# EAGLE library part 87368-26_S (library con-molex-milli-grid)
RECEPTACAL
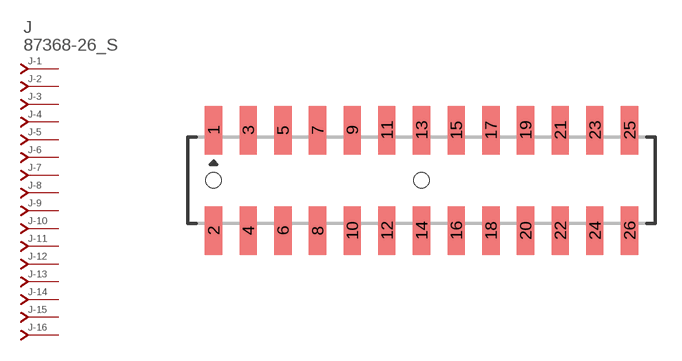
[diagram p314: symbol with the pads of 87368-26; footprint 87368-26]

Designator prefix J; gates -1=J-NV -2=J-N -3=J-N -4=J-N -5=J-N -6=J-N -7=J-N -8=J-N -9=J-N -10=J-N -11=J-N -12=J-N -13=J-N -14=J-N -15=J-N -16=J-N -17=J-N -18=J-N -19=J-N -20=J-N -21=J-N -22=J-N -23=J-N -24=J-N -25=J-N -26=J-N

## 87368-26_S  [87368-26]
1  -1:J  pas
2  -2:J  pas
3  -3:J  pas
4  -4:J  pas
5  -5:J  pas
6  -6:J  pas
7  -7:J  pas
8  -8:J  pas
9  -9:J  pas
10  -10:J  pas
11  -11:J  pas
12  -12:J  pas
13  -13:J  pas
14  -14:J  pas
15  -15:J  pas
16  -16:J  pas
17  -17:J  pas
18  -18:J  pas
19  -19:J  pas
20  -20:J  pas
21  -21:J  pas
22  -22:J  pas
23  -23:J  pas
24  -24:J  pas
25  -25:J  pas
26  -26:J  pas

## Footprint 87368-26 (pad centres in mm)
RECEPTACAL SMD Dual Row, Side Entry
smd 1 x 2.8: 1 -12,2.9; 2 -12,-2.9; 3 -10,2.9; 4 -10,-2.9; 5 -8,2.9; 6 -8,-2.9; 7 -6,2.9; 8 -6,-2.9; 9 -4,2.9; 10 -4,-2.9; 11 -2,2.9; 12 -2,-2.9; 13 0,2.9; 14 0,-2.9; 15 2,2.9; 16 2,-2.9; 17 4,2.9; 18 4,-2.9; 19 6,2.9; 20 6,-2.9; 21 8,2.9; 22 8,-2.9; 23 10,2.9; 24 10,-2.9; 25 12,2.9; 26 12,-2.9
hole 0.914 at -12,0
hole 0.914 at 0,0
